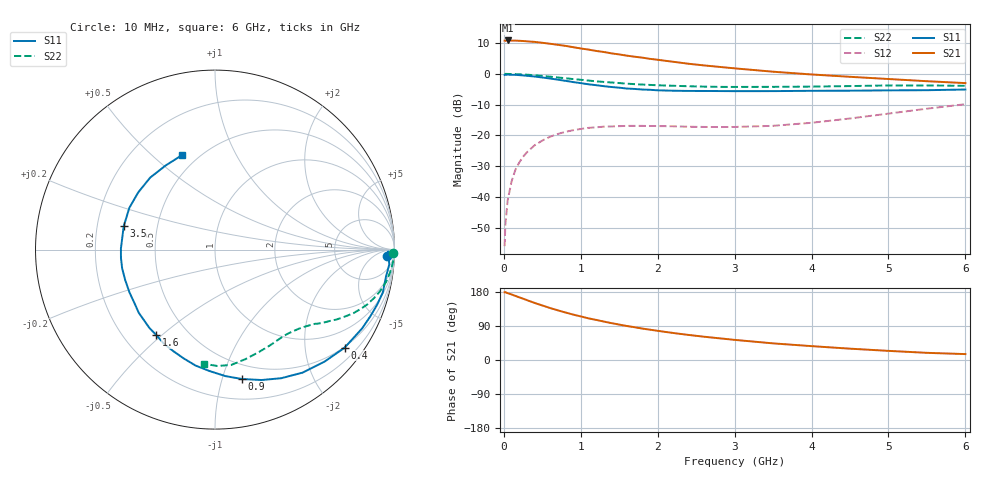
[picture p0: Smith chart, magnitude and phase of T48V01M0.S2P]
! Infineon Technologies  Discrete & RF Semiconductors
! BFR182T
! Si NPN RF Bipolar Junction Transistor in SC75
! VCE = 8 V  IC = 1 mA
! Common Emitter S-Parameters:  October  1999
# GHz  S  MA  R  50
!  f  S11  S21  S12  S22
! GHz  MAG  ANG  MAG  ANG  MAG  ANG  MAG  ANG
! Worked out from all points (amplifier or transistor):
!   36 points, 10 MHz to 6 GHz, reference 50 ohm
!   highest |S21| = 10.8 dB at 50 MHz (marker M1)
!   |S21| within 3 dB of that: start of sweep to 1.11 GHz
!   unconditionally stable (mu >= 1): 2.446 GHz to 4.612 GHz
!   at 250 MHz: K = 0.09, MSG = 18.8 dB, |S12| = -26.9 dB
!   at 1.4 GHz: K = 0.57, MSG = 11.9 dB, |S12| = -17.1 dB
!   at 6 GHz: K = 0.83, MSG = 3.4 dB, |S12| = -9.9 dB
!   S11 on the Smith chart (normalised r, x): 10 MHz: 28, -23; 400 MHz: 0.48, -2.91; 900 MHz: 0.37, -1.16; 1.6 GHz: 0.34, -0.48; 3.5 GHz: 0.32, +0.11; 6 GHz: 0.41, +0.63
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0.01  0.9588 -2.0  3.457 178.6  0.0016 78.8  0.9908 -1.2
0.02  0.9657 -0.6  3.443 178.9  0.0036 95.7  0.9999 -0.8
0.05  0.9744 -4.9  3.484 176.4  0.0089 92.1  0.9971 -1.9
0.1  0.9644 -9.1  3.461 173.0  0.0179 85.3  0.9949 -3.7
0.15  0.9651 -14.3  3.462 169.1  0.0277 81.6  0.9897 -5.5
0.25  0.9422 -23.1  3.412 161.8  0.0451 76.5  0.9767 -9.1
0.4  0.9057 -37.1  3.301 150.6  0.0693 68.4  0.9491 -14.1
0.5  0.873 -45.6  3.193 143.9  0.0828 63.3  0.926 -17.0
0.6  0.8412 -54.6  3.082 137.2  0.0954 59.0  0.9009 -19.9
0.7  0.8058 -62.8  2.963 131.2  0.1057 55.0  0.8746 -22.3
0.8  0.7714 -70.4  2.846 125.4  0.1146 51.1  0.8494 -24.6
0.9  0.7361 -78.3  2.711 119.9  0.1217 47.9  0.823 -26.6
1.1  0.6773 -92.6  2.479 109.9  0.1329 42.3  0.7785 -30.1
1.4  0.6117 -112.3  2.151 97.3  0.1402 35.9  0.7241 -34.3
1.6  0.5777 -124.5  1.973 89.7  0.1432 33.2  0.6937 -36.6
1.8  0.5573 -135.6  1.833 82.9  0.1431 31.6  0.6705 -39.2
2.2  0.5328 -153.4  1.572 71.3  0.141 30.7  0.641 -43.6
2.8  0.526 -174.9  1.298 57.3  0.137 34.6  0.6151 -51.3
3.5  0.5249 165.7  1.084 43.9  0.1435 44.7  0.6155 -60.3
4.5  0.5334 143.4  0.896 29.9  0.1888 57.5  0.6335 -74.5
5.5  0.5433 120.4  0.76 18.9  0.2723 60.2  0.6487 -88.8
6  0.5572 109.4  0.708 15.6  0.3217 58.0  0.639 -95.5
